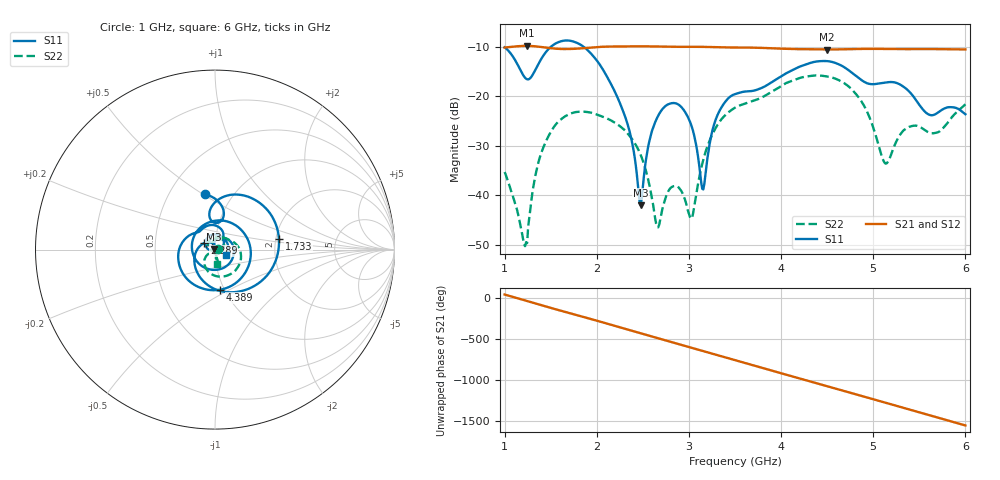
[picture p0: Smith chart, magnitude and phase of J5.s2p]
!Agilent Technologies,E8364B,MY43040528,A.07.50.67
!Agilent E8364B: A.07.50.67
!Date: Sunday, March 01, 2026 19:02:30
!Correction: S11(Full 2 Port(1,2))
!S21(Full 2 Port(1,2))
!S12(Full 2 Port(1,2))
!S22(Full 2 Port(1,2))
!S2P File: Measurements: S11, S21, S12, S22:
# Hz S  dB  R 50
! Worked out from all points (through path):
!   451 points, 1 GHz to 6 GHz, reference 50 ohm
!   highest |S21| = -9.78 dB at 1.244 GHz (marker M1); lowest = -10.5 dB at 4.5 GHz (marker M2)
!   group delay of S21, straight-line fit = 889 ps
!   lowest |S11| = -42.0 dB at 2.478 GHz (marker M3), VSWR 1.02, Z = 49.3 + j0.375 ohm
!   |S11| at or under -10 dB: start of sweep to 1.5 GHz; 1.859 GHz to end of sweep
!   |S22| runs from -50.3 to -15.8 dB; largest |S21 - S12| = 0.0015
!   S11 on the Smith chart (normalised r, x): 1 GHz: 0.74, +0.51; 1.733 GHz: 2.08, +0.30; 2.289 GHz: 0.89, +0.07; 4.389 GHz: 0.95, -0.45; 6 GHz: 1.12, -0.07
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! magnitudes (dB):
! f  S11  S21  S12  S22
! 1 GHz  -10.1  -10.1  -10.2  -35.3
! 1.244 GHz  -16.6  -9.8  -9.8  -49.7
! 1.411 GHz  -12.0  -10.1  -10.1  -30.8
! 1.733 GHz  -8.8  -10.4  -10.4  -23.4
! 1.844 GHz  -9.8  -10.3  -10.3  -23.1
! 2.289 GHz  -23.2  -9.9  -9.9  -26.6
! 2.478 GHz  -42.0  -9.9  -9.9  -31.9
! 2.667 GHz  -23.9  -9.9  -10.0  -46.5
! 2.8 GHz  -21.4  -10.0  -10.0  -38.6
! 2.956 GHz  -23.1  -10.0  -10.0  -40.8
! 3.033 GHz  -26.3  -10.0  -10.0  -44.6
! 3.156 GHz  -38.9  -10.0  -10.0  -32.8
! 3.289 GHz  -24.8  -10.0  -10.1  -26.5
! 3.5 GHz  -19.6  -10.1  -10.1  -22.3
! 4.344 GHz  -13.1  -10.5  -10.5  -15.8
! 4.389 GHz  -12.9  -10.5  -10.5  -15.8
! 4.5 GHz  -12.9  -10.5  -10.6  -16.0
! 4.844 GHz  -16.3  -10.4  -10.5  -20.3
! 5.167 GHz  -17.1  -10.4  -10.5  -33.0
! 5.344 GHz  -18.3  -10.4  -10.5  -26.7
! 5.6 GHz  -23.7  -10.4  -10.5  -27.3
! 6 GHz  -23.6  -10.5  -10.5  -21.6
